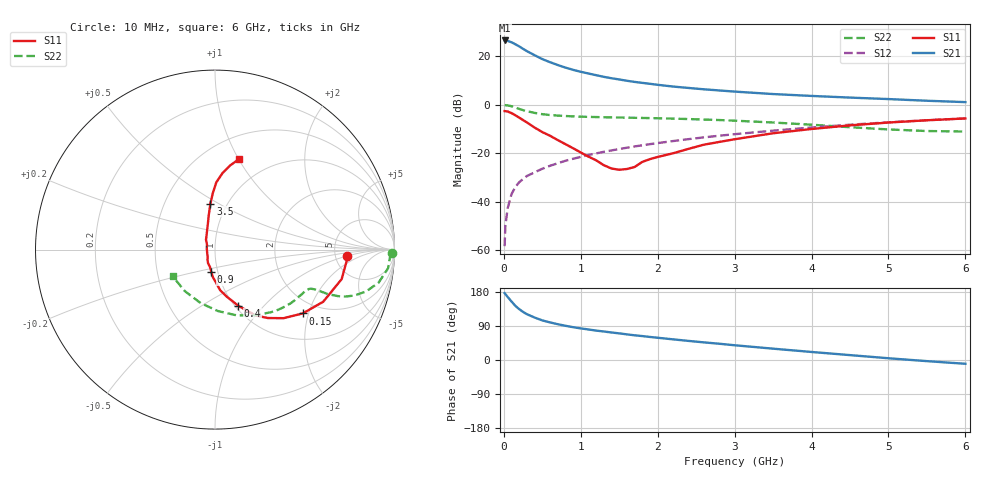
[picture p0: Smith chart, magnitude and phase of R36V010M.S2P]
! SIEMENS Small Signal Semiconductors
! BFR181
! Si NPN RF Bipolar Junction Transistor in SOT23
! VCE = 6 V  IC = 10 mA
! Common Emitter S-Parameters:  May  1996
# GHz  S  MA  R  50
!  f  S11  S21  S12  S22
! GHz  MAG  ANG  MAG  ANG  MAG  ANG  MAG  ANG
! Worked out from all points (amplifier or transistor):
!   36 points, 10 MHz to 6 GHz, reference 50 ohm
!   highest |S21| = 26.5 dB at 10 MHz (marker M1)
!   |S21| within 3 dB of that: start of sweep to 227.1 MHz
!   unconditionally stable (mu >= 1): 856.8 MHz to 2.714 GHz
!   at 250 MHz: K = 0.59, MSG = 26.9 dB, |S12| = -30.7 dB
!   at 1.4 GHz: K = 1.05, MAG = 13.5 dB, |S12| = -18.9 dB
!   at 6 GHz: K = 0.86, MSG = 3.4 dB, |S12| = -5.7 dB
!   S11 on the Smith chart (normalised r, x): 10 MHz: 6.50, -0.96; 150 MHz: 1.64, -1.84; 400 MHz: 1.03, -0.73; 900 MHz: 0.93, -0.24; 3.5 GHz: 0.84, +0.46; 6 GHz: 0.72, +1.00
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0.01  0.7384 -2.6  21.21 176.5  0.0012 93.9  0.9848 -1.1
0.02  0.7356 -5.2  20.84 173.9  0.0032 88.6  0.9757 -2.5
0.05  0.7247 -13.1  20.74 166.3  0.0073 83.7  0.9697 -6.2
0.1  0.6694 -25.7  19.45 154.3  0.0143 79.5  0.9293 -11.5
0.15  0.6049 -36.0  17.69 142.8  0.02 73.3  0.873 -15.5
0.2  0.5403 -45.0  15.99 134.2  0.0251 71.6  0.8187 -18.2
0.25  0.4819 -52.3  14.25 126.9  0.0293 69.7  0.7722 -19.8
0.3  0.4302 -58.5  12.75 120.9  0.0337 69.0  0.734 -20.7
0.4  0.3372 -67.6  10.51 112.0  0.0402 68.6  0.6774 -21.5
0.5  0.272 -75.7  8.752 104.5  0.0476 68.5  0.6375 -21.6
0.6  0.2286 -82.7  7.548 99.2  0.0548 69.1  0.6128 -21.6
0.7  0.1865 -87.9  6.61 94.5  0.0617 69.2  0.5962 -21.8
0.9  0.1262 -99.5  5.25 86.6  0.0766 69.6  0.5743 -22.3
1.1  0.0847 -117.3  4.409 80.6  0.0915 69.9  0.5605 -23.5
1.3  0.0563 -136.2  3.762 75.2  0.1065 69.3  0.551 -25.0
1.6  0.047 168.3  3.121 67.6  0.1296 68.1  0.5406 -28.1
2.2  0.0993 117.7  2.371 54.5  0.1776 65.0  0.5165 -35.5
2.6  0.1494 105.4  2.081 46.5  0.2116 62.0  0.4936 -41.5
3.5  0.2573 95.7  1.66 29.9  0.2912 54.3  0.4292 -58.6
4.5  0.3746 88.9  1.403 12.9  0.3864 43.7  0.3429 -87.2
5.5  0.4773 79.7  1.207 -3.0  0.4783 31.1  0.286 -125.9
6  0.5203 75.3  1.131 -10.0  0.5208 24.2  0.2792 -147.9
